ORGANIZATION_BLOCK "Cycle Time Fault"
TITLE =
VERSION : 0.1


VAR_TEMP
  OB80_EV_CLASS : BYTE ;	//16#35, Event class 3, Entering event state, Internal fault event
  OB80_FLT_ID : BYTE ;	//16#XX, Fault identifcation code
  OB80_PRIORITY : BYTE ;	//26 (Priority of 1 is lowest)
  OB80_OB_NUMBR : BYTE ;	//80 (Organization block 80, OB80)
  OB80_RESERVED_1 : BYTE ;	//Reserved for system
  OB80_RESERVED_2 : BYTE ;	//Reserved for system
  OB80_ERROR_INFO : WORD ;	//Error information on event
  OB80_ERR_EV_CLASS : BYTE ;	//Class of event causing error
  OB80_ERR_EV_NUM : BYTE ;	//Number of event causing error
  OB80_OB_PRIORITY : BYTE ;	//Priority of OB causing error
  OB80_OB_NUM : BYTE ;	//Number of OB causing error
  OB80_DATE_TIME : DATE_AND_TIME ;	//Date and time OB80 started
END_VAR
BEGIN
END_ORGANIZATION_BLOCK

